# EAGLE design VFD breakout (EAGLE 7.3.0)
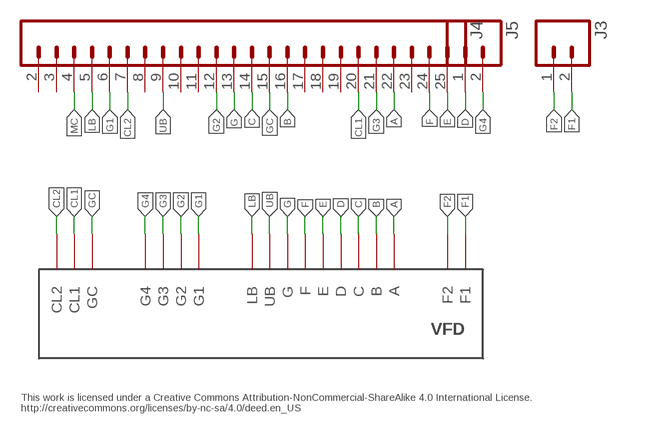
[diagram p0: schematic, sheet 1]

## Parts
J3  M02PTH  [1X02]
J4  M24  [1X24]
J5  M02PTH  [1X02]
U$1  VFD_5LT43  [VFD_5LT43]

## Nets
A: J4.22 U$1.A
B: J4.16 U$1.B
C: J4.14 U$1.C
CL1: J4.20 U$1.CL1
CL2: J4.7 U$1.CL2
D: J5.1 U$1.D
E: J4.25 U$1.E
F: J4.24 U$1.F
F1: J3.2 U$1.F1
F2: J3.1 U$1.F2
G: J4.13 U$1.G
G1: J4.6 U$1.G1
G2: J4.12 U$1.G2
G3: J4.21 U$1.G3
G4: J5.2 U$1.G4
GC: J4.15 U$1.GC
LB: J4.5 U$1.LB
MC: J4.4
UB: J4.9 U$1.UB
Unconnected: J4.2 J4.3 J4.8 J4.10 J4.11 J4.17 J4.18 J4.19 J4.23

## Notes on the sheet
- This work is licensed under a Creative Commons Attribution-NonCommercial-ShareAlike 4.0 International License.
  http://creativecommons.org/licenses/by-nc-sa/4.0/deed.en_US

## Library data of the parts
J3 J5 = SparkFun-Connectors:M02: Standard 2-pin 0.1" header. Use with
J4 = SparkFun-Connectors:M24: 1x24 .1" header
U$1 = VFD_5LT43:VFD_5LT43: Futaba 5LT43 VFD Filament: 2.7 - 3.3 Vac, 3.0V recommended Anode/Grid: 34Vp-p max, 26V recommended

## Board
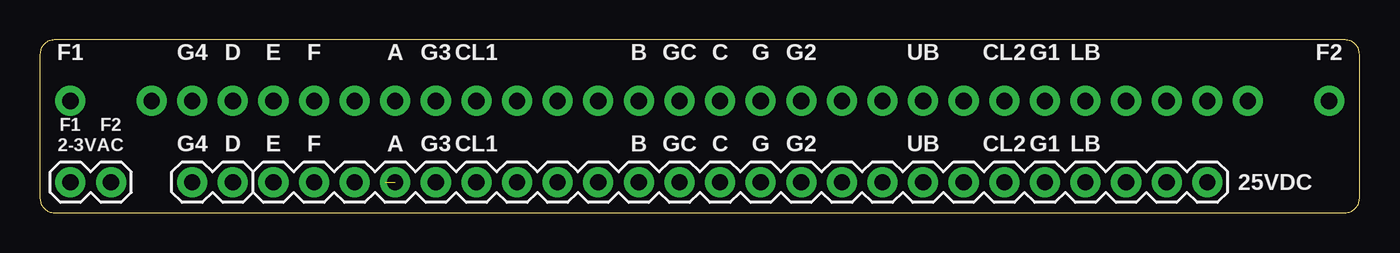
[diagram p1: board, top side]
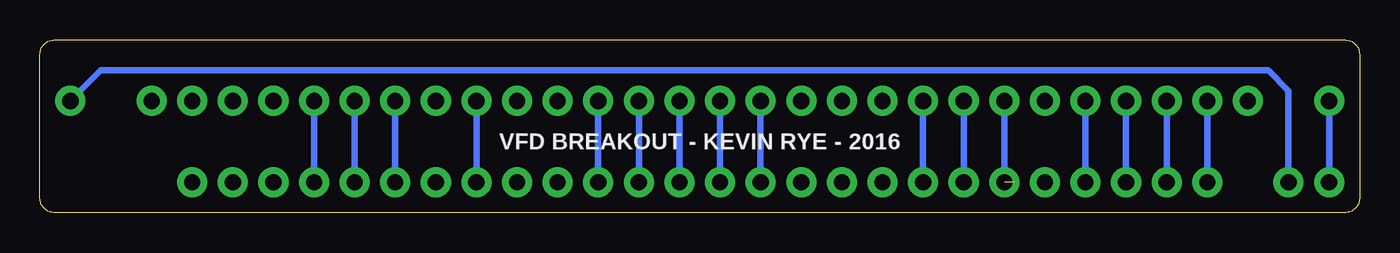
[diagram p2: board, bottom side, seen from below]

Size 82.55 x 10.79 mm. Coordinates in mm from the lower left corner, seen from the top.
Outline: 82.55,0.9 82.55,9.9 arc90 81.65,10.79 0.9,10.79 arc90 0,9.9 0,0.9 arc90 0.9,0 81.65,0 arc90 82.55,0.9
Copper layers (1*16): Top 0.035mm / dielectric 1.5mm / Bottom 0.035mm
Design rules "default": minimum track width 10mil, minimum drill 24mil, track to track 8mil, track to pad 8mil, pad to pad 8mil, via to via 8mil, smd to smd 8mil, copper to edge 40mil, drill to drill 8mil, minimum pad ring 10mil, minimum via ring 8mil, stop-mask expansion 4mil, vias tented up to drill 0mil, thermal gap 10mil

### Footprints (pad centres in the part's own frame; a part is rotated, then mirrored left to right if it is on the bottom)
1X02 = drill 1.016 pad 1.88: 1 0,0; 2 2.54,0
1X24 = drill 1.016 pad 1.88: 2 -26.67,0; 3 -24.13,0; 4 -21.59,0; 5 -19.05,0; 6 -16.51,0; 7 -13.97,0; 8 -11.43,0; 9 -8.89,0; 10 -6.35,0; 11 -3.81,0; 12 -1.27,0; 13 1.27,0; 14 3.81,0; 15 6.35,0; 16 8.89,0; 17 11.43,0; 18 13.97,0; 19 16.51,0; 20 19.05,0; 21 21.59,0; 22 24.13,0; 23 26.67,0; 24 29.21,0; 25 31.75,0
VFD_5LT43 = drill 1.016 pad 1.88: 3 7.62,0; 12 30.48,0; 13 33.02,0; 20 50.8,0; 21 53.34,0; 28 71.12,0; 30 76.2,0; A 22.86,0; B 38.1,0; C 43.18,0; CL1 27.94,0; CL2 60.96,0; D 12.7,0; E 15.24,0; F 17.78,0; F1 2.54,0; F2 81.28,0; G 45.72,0; G1 63.5,0; G1_1 73.66,0; G2 48.26,0; G2_1 58.42,0; G3 25.4,0; G3_1 35.56,0; G4 10.16,0; G4_1 20.32,0; GC 40.64,0; LB 66.04,0; MC 68.58,0; UB 55.88,0

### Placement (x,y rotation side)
J3  4.45,1.91 180 top
J4  46.35,1.91 180 top
J5  12.06,1.91 180 top
U$1  -0.64,6.99 0 top

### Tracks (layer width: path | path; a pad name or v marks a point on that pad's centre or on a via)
A  (1 unrouted)
  Bottom 0.406: U$1.A 22.23,2.54 21.59,1.91
B
  Bottom 0.406: U$1.B J4.16
C
  Bottom 0.406: U$1.C J4.14
CL1
  Bottom 0.406: U$1.CL1 J4.20
CL2
  Bottom 0.406: U$1.CL2 J4.7
D
  Bottom 0.406: U$1.D J5.1
E
  Bottom 0.406: U$1.E J4.25
F
  Bottom 0.406: U$1.F J4.24
F1
  Bottom 0.406: U$1.F1 J3.2
F2
  Bottom 0.406: J3.1 4.45,7.62 5.71,8.89 78.74,8.89 U$1.F2
G
  Bottom 0.406: U$1.G J4.13
G1
  Bottom 0.406: U$1.G1 J4.6
G2
  Bottom 0.406: U$1.G2 J4.12
G3
  Bottom 0.406: J4.21 U$1.G3
G4
  Bottom 0.406: J5.2 U$1.G4
GC
  Bottom 0.406: U$1.GC J4.15
LB
  Bottom 0.406: U$1.LB J4.5
UB
  Bottom 0.406: U$1.UB J4.9

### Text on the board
Unrouted: This work is licensed under a Creative Commons Attribution-NonCommercial-ShareAlike 4.0 International License. / http://creativecommons.org/licenses/by-nc-sa/4.0/deed.en_US
tNames: F1 | F2 | 2-3VAC | G4 | D | E | F | A | G3 | CL1 | B | GC | C | G | G2 | UB | CL2 | G1 | LB | 25VDC
bNames: VFD BREAKOUT - KEVIN RYE - 2016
